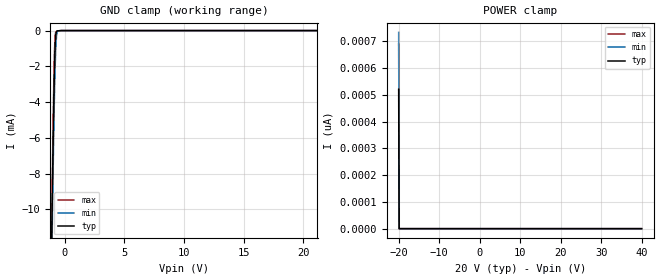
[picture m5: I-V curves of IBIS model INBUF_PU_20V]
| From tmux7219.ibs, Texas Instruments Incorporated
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| Model10
[Model]   INBUF_PU_20V
Model_type   Input
Vinl = 0.8
Vinh = 1.3
|   typ   min   max
C_comp   1.85pF   1.7pF   2.1pF
[Voltage Range]   20   18   22
[Temperature Range]   27   125   -40
[Power Clamp Reference]   20   18   22
[GND Clamp Reference]   0   0   0
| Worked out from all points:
|   GND clamp passes 1 mA (typ) near -0.80 V on its own axis
[GND Clamp]
|   Voltage   I(typ)   I(min)   I(max)
-20V      -1.029A    -1.028A    -1.031A
-1.1V     -12.66mA   -14mA      -11.59mA
-1.04V    -9.827mA   -11.25mA   -8.704mA
-980mV    -7.116mA   -8.605mA   -5.939mA
-920mV    -4.606mA   -6.142mA   -3.408mA
-860mV    -2.464mA   -3.96mA    -1.379mA
-800mV    -957.3uA   -2.208mA   -298.3uA
-740mV    -229.8uA   -1.002mA   -69.73uA
-680mV    -49.95uA   -330.4uA   -42.8uA
-620mV    -21.95uA   -80.57uA   -30.72uA
-320mV    -737.7nA   -856.8nA   -877.7nA
40V       0A         0A         0A
[POWER Clamp]
|   Voltage   I(typ)   I(min)   I(max)
-20V      520.3pA    732.7pA    690.3pA
-19.88V   0A         0A         0A
-19.82V   0A         0A         0A
40V       0A         0A         0A
